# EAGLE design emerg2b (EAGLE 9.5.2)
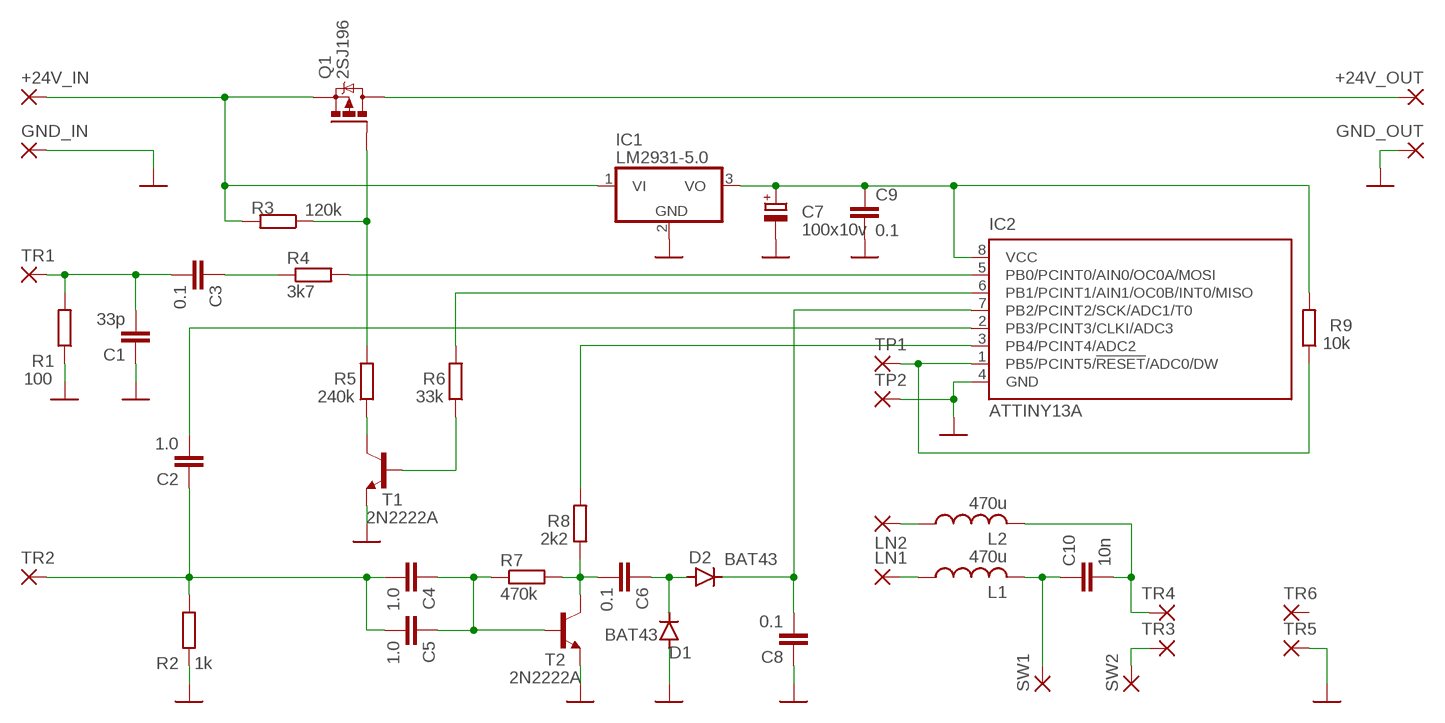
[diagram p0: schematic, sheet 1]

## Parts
+24V_IN  3,17/1,3  [3,17/1,3]
+24V_OUT  3,17/1,3  [3,17/1,3]
C1  33p  C-EU025-025X050  [C025-025X050]
C2  1.0  C-EU050-025X075  [C050-025X075]
C3  0.1  C-EU025-025X050  [C025-025X050]
C4  1.0  C-EU050-025X075  [C050-025X075]
C5  1.0  C-EU050-025X075  [C050-025X075]
C6  0.1  C-EU025-025X050  [C025-025X050]
C7  100x10v  CPOL-EUE2.5-5  [E2,5-5]
C8  0.1  C-EU025-025X050  [C025-025X050]
C9  0.1  C-EU025-025X050  [C025-025X050]
C10  10n  C-EU075-032X103  [C075-032X103]
D1  BAT43  1N4148DO35-10  [DO35-10]
D2  BAT43  1N4148DO35-7  [DO35-7]
GND_IN  3,17/1,3  [3,17/1,3]
GND_OUT  3,17/1,3  [3,17/1,3]
IC1  LM2931-5.0  7805TV  [TO220V]
IC2  ATTINY13A  TINY13-20PU  [DIL08]
L1  470u  L-US6000-XXX-RC  [6000-XXXX-RC]
L2  470u  L-US6000-XXX-RC  [6000-XXXX-RC]
LN1  3,17/1,3  [3,17/1,3]
LN2  3,17/1,3  [3,17/1,3]
Q1  2SJ196  IRF9530  [TO220BV]
R1  100  R-EU_0204/2V  [0204V]
R2  1k  R-EU_0204/7  [0204/7]
R3  120k  R-EU_0204/7  [0204/7]
R4  3k7  R-EU_0204/7  [0204/7]
R5  240k  R-EU_0204/2V  [0204V]
R6  33k  R-EU_0204/2V  [0204V]
R7  470k  R-EU_0204/2V  [0204V]
R8  2k2  R-EU_0204/7  [0204/7]
R9  10k  R-EU_0204/7  [0204/7]
SW1  3,17/1,3  [3,17/1,3]
SW2  3,17/1,3  [3,17/1,3]
T1  2N2222A  2N2222  [TO92-EBC-OVAL]
T2  2N2222A  2N2222  [TO92-EBC-OVAL]
TP1  2,15/1,0  [2,15/1,0]
TP2  2,15/1,0  [2,15/1,0]
TR1  2,15/1,0  [2,15/1,0]
TR2  2,15/1,0  [2,15/1,0]
TR3  2,15/1,0  [2,15/1,0]
TR4  2,15/1,0  [2,15/1,0]
TR5  2,15/1,0  [2,15/1,0]
TR6  2,15/1,0  [2,15/1,0]

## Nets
GND: C1.1 C7.- C8.1 C9.2 D1.A GND_IN.1(P) GND_OUT.1(P) IC1.2(GND) IC2.4(GND) R1.1 R2.1 T1.E T2.E TP2.1(P) TR5.1(P)
N$1: C6.1 D1.C D2.A
N$2: C6.2 R7.2 R8.1 T2.C
N$3: R5.1 T1.C
N$4: IC2.6(PB1/PCINT1/AIN1/OC0B/INT0/MISO) R6.2
N$5: C4.1 C5.1 R7.1 T2.B
N$6: IC2.3(PB4/PCINT4/ADC2) R8.2
N$7: IC2.1(PB5/PCINT5/!RESET!/ADC0/DW) R9.1 TP1.1(P)
N$8: C2.1 C4.2 C5.2 R2.2 TR2.1(P)
N$9: C8.2 D2.C IC2.7(PB2/PCINT2/SCK/ADC1/T0)
N$10: C7.+ C9.1 IC1.3(VO) IC2.8(VCC) R9.2
N$11: C3.1 R4.1
N$12: C1.2 C3.2 R1.2 TR1.1(P)
N$13: C2.2 IC2.2(PB3/PCINT3/CLKI/ADC3)
N$14: IC2.5(PB0/PCINT0/AIN0/OC0A/MOSI) R4.2
N$15: +24V_IN.1(P) IC1.1(VI) Q1.S R3.2
N$16: Q1.G R3.1 R5.2
N$17: +24V_OUT.1(P) Q1.D
N$18: R6.1 T1.B
N$19: C10.1 L1.2 SW1.1(P)
N$20: C10.2 L2.2 TR4.1(P)
N$21: SW2.1(P) TR3.1(P)
N$22: L2.1 LN2.1(P)
N$23: L1.1 LN1.1(P)
Unconnected: TR6.1(P)

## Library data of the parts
+24V_IN +24V_OUT GND_IN GND_OUT LN1 LN2 SW1 SW2 = wirepad:3,17/1,3: THROUGH-HOLE PAD
C1-C6 C8-C10 = rcl:C-EU: CAPACITOR, European symbol; SPICEPREFIX: C
C7 = rcl:CPOL-EU: POLARIZED CAPACITOR, European symbol
D1 D2 = diode:1N4148: DIODE
IC1 = linear:78*: Positive VOLTAGE REGULATOR Source: http://cache.national.com/ds/LM/LM78L05.pdf http://www.fairchildsemi.com/ds/LM/LM7805.pdf
IC2 = atmel:TINY13: 8-bit AVR Microcontroller with 1K Bytes In-System Programmable Flash Source: http://www.atmel.com/dyn/resources/prod_documents/2535S.pdf; MPN: ATTINY13-20PU; OC_FARNELL: 9171550; OC_NEWARK: 96K6521
L1 L2 = rcl:L-US: INDUCTOR, American symbol; SPICEPREFIX: L
Q1 = transistor-power:IRF9530: P-CHANNEL HEXFET POWER-MOS-FET Source: http://www.irf.com/product-info/datasheets/data/irf9530.pdf
R1-R9 = rcl:R-EU_: RESISTOR, European symbol; SPICEPREFIX: R
T1 T2 = adafruit:2N2222: NPN TRANSISTOR Big oval pads
TP1 TP2 TR1-TR6 = wirepad:2,15/1,0: THROUGH-HOLE PAD

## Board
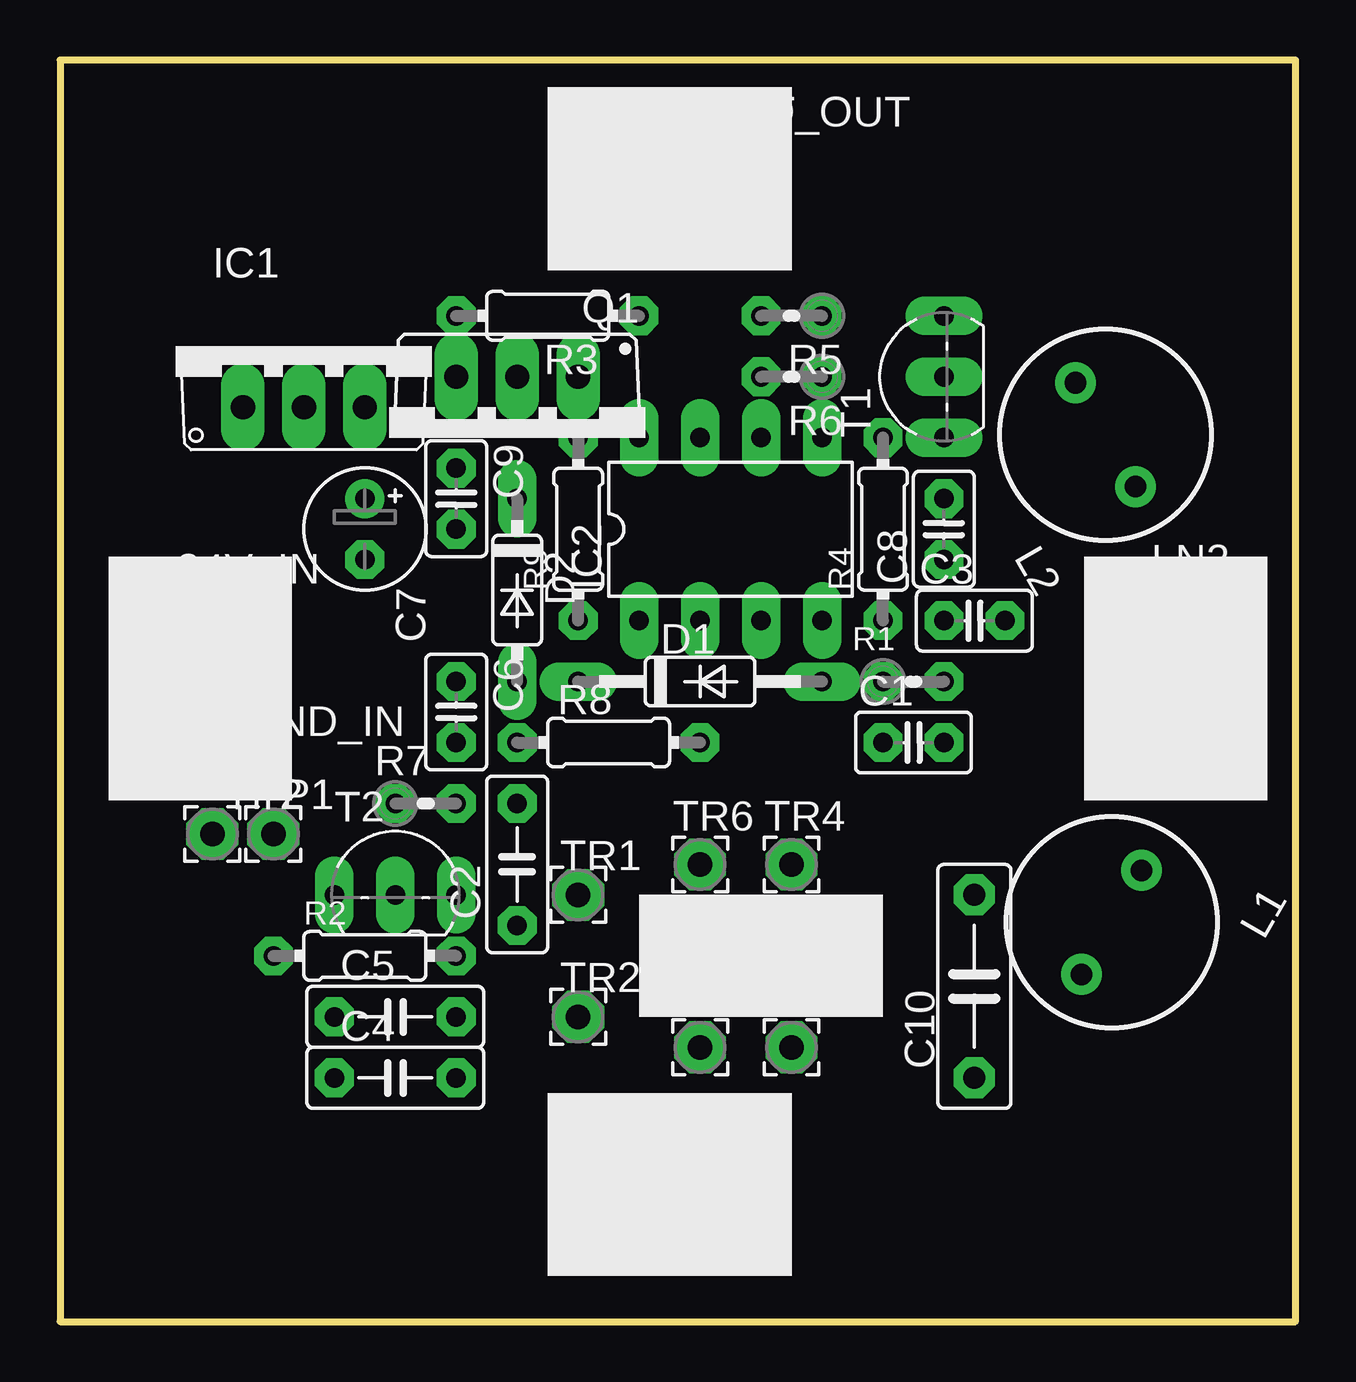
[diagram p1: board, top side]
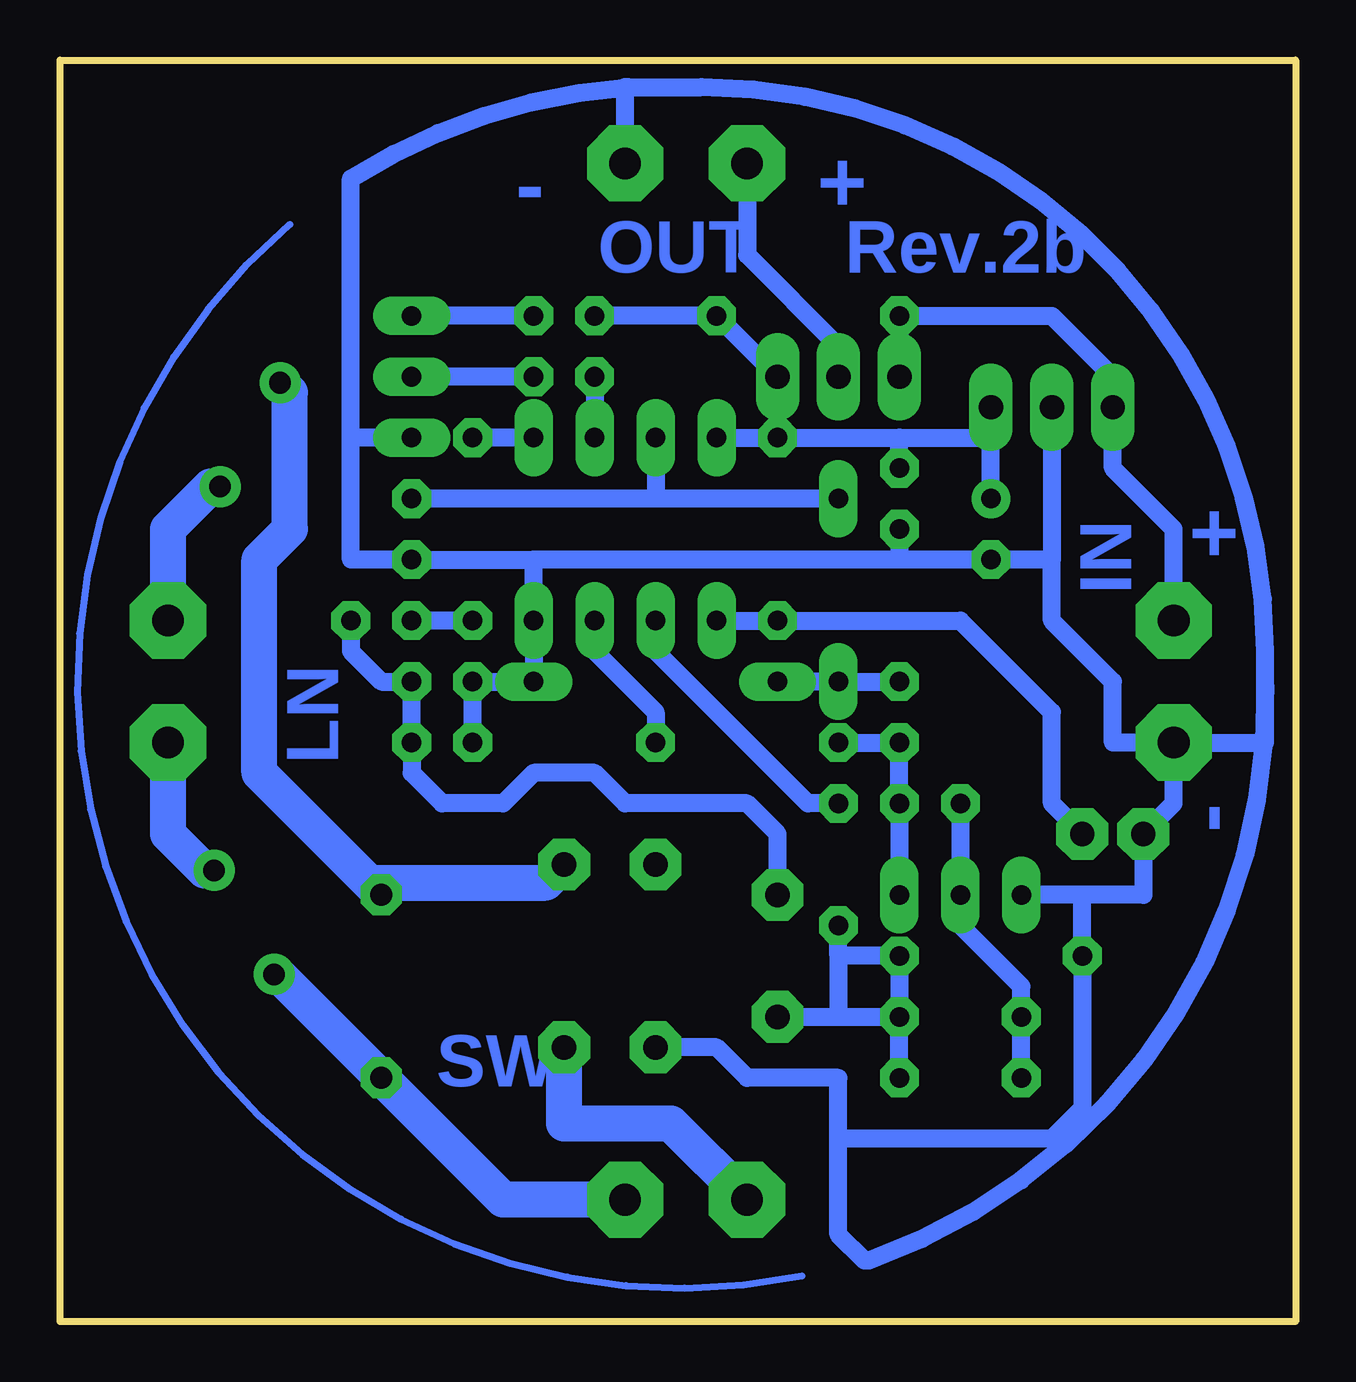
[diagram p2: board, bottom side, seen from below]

Size 51.49 x 52.57 mm. Coordinates in mm from the lower left corner, seen from the top.
Outline: 0,0 51.49,0 51.49,52.57 0,52.57 0,0
Copper layers (1*16): Top 0.035mm / dielectric 1.5mm / Bottom 0.035mm
Design rules "fab_board": minimum track width 0.3mm, minimum drill 0.6mm, track to track 0.15mm, track to pad 0.15mm, pad to pad 0.15mm, via to via 0.15mm, smd to smd 0.15mm, copper to edge 0.15mm, drill to drill 0.15mm, minimum pad ring 0.4mm, minimum via ring 0.5mm, stop-mask expansion 4mil, vias tented up to drill 0mil, thermal gap 0.5mm

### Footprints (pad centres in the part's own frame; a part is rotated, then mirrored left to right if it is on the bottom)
3,17/1,3 = drill 1.321 pad 3.175 octagon: 1 0,0
C025-025X050 = drill 0.813 octagon: 1 -1.27,0; 2 1.27,0
C050-025X075 = drill 0.813 octagon: 1 -2.54,0; 2 2.54,0
E2,5-5 = drill 0.813 pad 1.6: + -1.27,0 | drill 0.813 pad 1.6 octagon: - 1.27,0
C075-032X103 = drill 0.914 octagon: 1 -3.81,0; 2 3.81,0
DO35-10 = drill 0.813 long: A 5.08,0; C -5.08,0
DO35-7 = drill 0.813 long: A 3.81,0; C -3.81,0
TO220V = drill 1.016 long: 1 -2.54,-2.54; 2 0,-2.54; 3 2.54,-2.54
DIL08 = drill 0.813 long: 1 -3.81,-3.81; 2 -1.27,-3.81; 3 1.27,-3.81; 4 3.81,-3.81; 5 3.81,3.81; 6 1.27,3.81; 7 -1.27,3.81; 8 -3.81,3.81
6000-XXXX-RC = drill 0.9 pad 1.422: 1 -2.5,0; 2 2.5,0
TO220BV = drill 1.016 long: D 0,-2.54; G -2.54,-2.54; S 2.54,-2.54
0204V = drill 0.813 octagon: 1 -1.27,0; 2 1.27,0
0204/7 = drill 0.813 octagon: 1 -3.81,0; 2 3.81,0
TO92-EBC-OVAL = drill 0.813 long: B 0,-1.27; C 2.54,-1.27; E -2.54,-1.27
2,15/1,0 = drill 1.016 pad 2.159 octagon: 1 0,0

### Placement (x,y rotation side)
+24V_IN  5.08,29.21 0 top
+24V_OUT  22.86,48.26 0 top
C1  35.56,24.13 0 top
C2  19.05,19.05 90 top
C3  38.1,29.21 0 top
C4  13.97,10.16 0 top
C5  13.97,12.7 0 top
C6  16.51,25.4 270 top
C7  12.7,33.02 270 top
C8  36.83,33.02 90 top
C9  16.51,34.29 270 top
C10  38.1,13.97 90 top
D1  26.67,26.67 0 top
D2  19.05,30.48 270 top
GND_IN  5.08,24.13 0 top
GND_OUT  27.94,48.26 0 top
IC1  10.16,40.64 0 top
IC2  27.94,33.02 0 top
L1  43.81,16.64 240 top
L2  43.56,36.96 120 top
LN1  46.99,24.13 0 top
LN2  46.99,29.21 0 top
Q1  19.05,36.83 180 top
R1  35.56,26.67 0 top
R2  12.7,15.24 0 top
R3  20.32,41.91 180 top
R4  34.29,33.02 90 top
R5  30.48,41.91 180 top
R6  30.48,39.37 180 top
R7  15.24,21.59 0 top
R8  22.86,24.13 0 top
R9  21.59,33.02 90 top
SW1  27.94,5.08 0 top
SW2  22.86,5.08 0 top
T1  35.56,39.37 90 top
T2  13.97,19.05 0 top
TP1  8.89,20.32 0 top
TP2  6.35,20.32 0 top
TR1  21.59,17.78 0 top
TR2  21.59,12.7 0 top
TR3  30.48,11.43 0 top
TR4  30.48,19.05 0 top
TR5  26.67,11.43 0 top
TR6  26.67,19.05 0 top

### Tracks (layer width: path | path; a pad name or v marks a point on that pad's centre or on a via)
GND
  Bottom 0.75: IC1.2 10.16,31.75 | 31.75,31.75 IC2.4 D1.A R1.1 C1.1 | 10.16,31.75 C7.- 16.51,31.75 | 31.75,31.75 C8.1 39.37,31.75 39.37,36.83 | 16.51,31.75 31.75,31.75 | C9.2 16.51,31.75 | 10.16,31.75 10.16,29.21 7.62,26.67 7.62,24.13 GND_IN.1 | T1.E 39.37,36.83 | GND_IN.1 5.08,21.59 TP2.1 6.35,17.78 8.89,17.78 | 8.89,17.78 T2.E | 1.27,26.54 arc72 17.78,2.54 17.96,2.54 19.05,3.62 19.05,7.62 | GND_IN.1 1.27,24.13 1.27,26.54 | GND_OUT.1 27.94,51.44 27.81,51.44 | 27.81,51.44 24.77,51.44 arc90 1.27,27.94 1.27,26.54 | 19.05,7.62 19.05,10.16 22.86,10.16 24.13,11.43 TR5.1 | 27.81,51.44 arc-28 39.37,47.62 39.37,36.83 | 8.89,17.78 R2.1 8.89,8.89 10.16,7.62 19.05,7.62
N$1
  Bottom 0.75: D1.C D2.A C6.1
N$2
  Bottom 0.75: R8.1 C6.2 R7.2 T2.C
N$3
  Bottom 0.75: R5.1 T1.C
N$4
  Bottom 0.75: R6.2 IC2.6
N$5
  Bottom 0.75: R7.1 T2.B 13.97,16.51 11.43,13.97 C5.1 C4.1
N$6
  Bottom 0.75: IC2.3 29.21,27.94 26.67,25.4 R8.2
N$7
  Bottom 0.75: TP1.1 10.16,21.59 10.16,25.4 13.97,29.21 R9.1 IC2.1
N$8
  Bottom 0.75: C5.2 R2.2 19.05,15.24 | C4.2 C5.2 | 19.05,15.24 C2.1 | TR2.1 19.05,12.7 | 19.05,12.7 C5.2 | 19.05,15.24 19.05,12.7
N$9
  Bottom 0.75: IC2.7 26.67,34.29 | 26.67,34.29 C8.2 | D2.C 26.67,34.29
N$10
  Bottom 0.75: IC2.8 R9.2 16.51,36.83 | 16.51,36.83 12.7,36.83 | C7.+ 12.7,36.83 | 12.7,36.83 IC1.3 | C9.1 16.51,36.83
N$11
  Bottom 0.75: R4.1 C3.1
N$12
  Bottom 0.75: C3.2 39.37,27.94 38.1,26.67 R1.2 C1.2 36.83,22.86 35.56,21.59 33.02,21.59 31.75,22.86 29.21,22.86 27.94,21.59 22.86,21.59 21.59,20.32 TR1.1
N$13
  Bottom 0.75: C2.2 20.32,21.59 26.67,27.94 IC2.2
N$14
  Bottom 0.75: IC2.5 R4.2
N$15
  Bottom 0.75: Q1.S R3.2 10.16,41.91 7.62,39.37 IC1.1 7.62,35.56 5.08,33.02 +24V_IN.1
N$16
  Bottom 0.75: Q1.G R3.1 R5.2
N$17
  Bottom 0.75: +24V_OUT.1 22.86,44.45 19.05,40.64 Q1.D
N$18
  Bottom 0.75: R6.1 T1.B
N$19
  Bottom 1.5: SW1.1 33.02,5.08 C10.1 42.41,14.47 L1.2
N$20
  Bottom 1.5: 38.61,18.29 31.24,18.29 TR4.1 | 38.61,18.29 43.18,22.86 43.18,31.75 41.91,33.02 41.91,38.72 L2.2 | 38.61,18.29 C10.2
N$21
  Bottom 1.5: SW2.1 26.04,8.25 30.48,8.25 TR3.1
N$22
  Bottom 1.5: L2.1 45.22,34.79 46.99,33.02 LN2.1
N$23
  Bottom 1.5: LN1.1 46.99,20.32 45.47,18.8 L1.1
N$24
  Bottom 0.3: 41.91,45.72 arc-151 20.57,1.91

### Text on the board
Bottom: + | - | Rev.2b | OUT | IN | + | LN | - | SW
